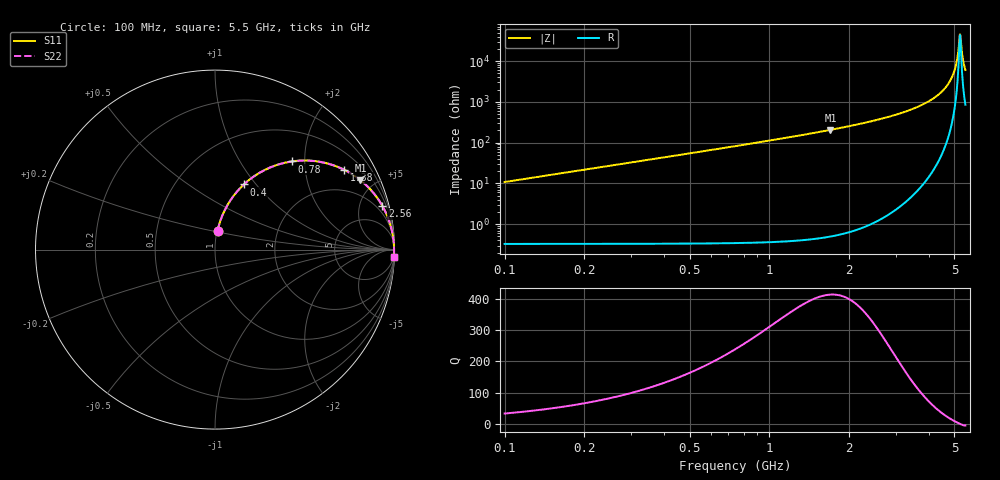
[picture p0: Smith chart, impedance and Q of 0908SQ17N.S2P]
! Coilcraft 0908SQ-17N Air Core Inductor
! 06 March 2008
# MHZ S MA R 50
!Freq  MagS11  AngS11  MagS21  AngS21  MagS12  AngS12  MagS22  AngS22
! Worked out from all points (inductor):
!   271 points, 100 MHz to 5.5 GHz, reference 50 ohm
!   read as one part in series: L = 17.2 nH near 120 MHz
!   highest Q = 413 at 1.7 GHz (marker M1), where L = 19.2 nH
!   self-resonance near 5.24 GHz
!   S11 on the Smith chart (normalised r, x): 100 MHz: 1.01, +0.22; 400 MHz: 1.01, +0.87; 780 MHz: 1.01, +1.73; 1.38 GHz: 1.03, +3.23; 2.56 GHz: 1.12, +7.59; 5.5 GHz: 3, -46
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100  0.107 82.1  0.991 -6.2  0.991 -6.2  0.107 82.1
160  0.1698 79.1  0.9823 -9.8  0.9823 -9.8  0.1698 79.1
220  0.2306 75.8  0.9698 -13.4  0.9698 -13.4  0.2307 75.8
400  0.3971 66.1  0.9147 -23.5  0.9147 -23.5  0.3971 66.1
780  0.651 48.9  0.7564 -40.8  0.7564 -40.8  0.6511 48.9
1000  0.7447 41.4  0.665 -48.4  0.665 -48.4  0.7447 41.4
1380  0.847 31.6  0.5294 -58.3  0.5294 -58.3  0.847 31.6
1700  0.8979 25.5  0.438 -64.3  0.438 -64.3  0.8979 25.5
1900  0.9199 22.4  0.3898 -67.4  0.3898 -67.4  0.92 22.4
2560  0.9632 14.7  0.2656 -75.1  0.2656 -75.1  0.9632 14.7
2800  0.9723 12.5  0.23 -77.2  0.23 -77.2  0.9723 12.5
3700  0.991 6.1  0.1247 -83.3  0.1247 -83.3  0.991 6.1
4220  0.9955 3.3  0.0772 -85.7  0.0772 -85.7  0.9956 3.3
4600  0.9972 1.4  0.04657 -86.5  0.04657 -86.5  0.9972 1.4
4860  0.9978 0.2  0.0272 -85.9  0.0272 -85.9  0.9978 0.2
5040  0.9979 -0.6  0.01448 -82.8  0.01448 -82.8  0.9979 -0.6
5160  0.9979 -1.1  0.006424 -72.4  0.006424 -72.4  0.9979 -1.1
5240  0.9979 -1.4  0.002223 -19.4  0.002223 -19.4  0.9979 -1.4
5260  0.9979 -1.5  0.002226 15.5  0.002226 15.5  0.9979 -1.5
5320  0.9978 -1.7  0.005113 63.1  0.005113 63.1  0.9978 -1.7
5360  0.9978 -1.9  0.007583 71.2  0.007583 71.2  0.9978 -1.9
5500  0.9975 -2.5  0.01646 79.5  0.01646 79.5  0.9976 -2.5
